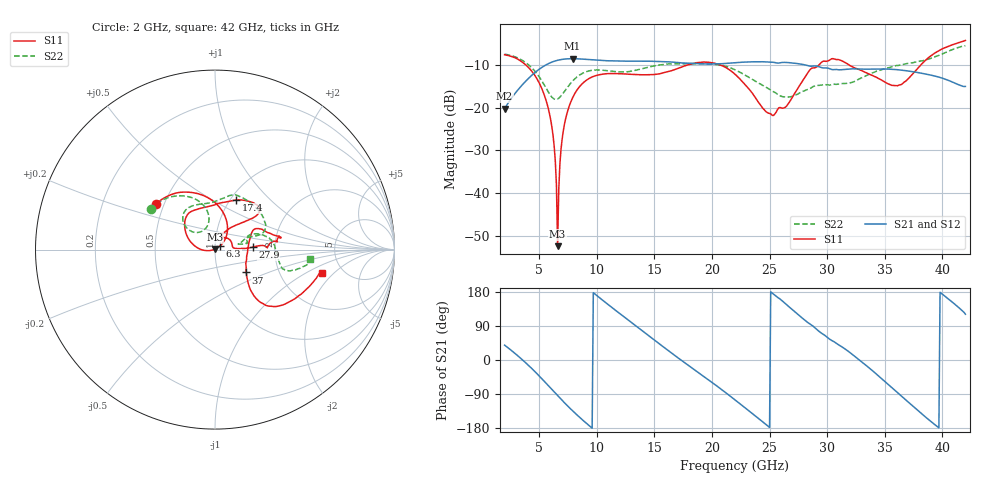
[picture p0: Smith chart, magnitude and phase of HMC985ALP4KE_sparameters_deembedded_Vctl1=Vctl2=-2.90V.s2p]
!s2p File: Measurements: S11, S21, S12, S22
# GHz S dB R 50.0
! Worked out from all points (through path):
!   401 points, 2 GHz to 42 GHz, reference 50 ohm
!   highest |S21| = -8.54 dB at 7.9 GHz (marker M1); lowest = -20.2 dB at 2 GHz (marker M2)
!   lowest |S11| = -52.4 dB at 6.6 GHz (marker M3), VSWR 1.00, Z = 50 + j0.238 ohm
!   |S11| at or under -10 dB: 3.839 GHz to 17.88 GHz (14.05 GHz wide, 129 % of centre); 20.69 GHz to 29.29 GHz (8.598 GHz wide, 34.4 % of centre); 31.9 GHz to 38.13 GHz (6.234 GHz wide, 17.8 % of centre)
!   |S22| runs from -18.1 to -5.5 dB; largest |S21 - S12| = 0.0006
!   S11 on the Smith chart (normalised r, x): 2 GHz: 0.45, +0.28; 6.3 GHz: 1.06, +0.04; 17.4 GHz: 1.06, +0.65; 27.9 GHz: 1.53, +0.04; 37 GHz: 1.36, -0.36; 42 GHz: 3.49, -1.46
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2  -7.62 142.5  -20.23 39.2  -20.22 39.2  -7.48 148.0
5  -14.20 73.6  -11.01 -42.1  -11.00 -42.1  -12.78 102.2
5.8  -20.27 49.5  -9.70 -67.8  -9.70 -67.8  -16.36 103.8
6.3  -28.93 36.4  -9.15 -84.2  -9.16 -84.2  -17.97 117.3
6.4  -32.43 34.9  -9.06 -87.4  -9.07 -87.4  -18.07 120.8
6.6  -52.40 96.2  -8.91 -93.9  -8.93 -93.9  -17.98 127.7
6.8  -33.14 -169.4  -8.80 -100.3  -8.81 -100.3  -17.53 133.7
7.1  -25.34 -174.7  -8.66 -109.8  -8.67 -109.8  -16.54 139.8
7.9  -17.70 165.5  -8.54 -134.0  -8.54 -134.0  -13.78 142.2
8.7  -14.50 149.8  -8.63 -156.4  -8.63 -156.4  -12.06 136.1
12.3  -12.08 118.3  -9.11 115.4  -9.11 115.4  -11.65 97.5
15.4  -12.11 91.4  -9.20 43.3  -9.19 43.3  -10.03 73.8
17.4  -10.46 67.1  -9.53 -1.8  -9.54 -1.8  -9.72 64.1
22  -12.16 41.7  -9.48 -105.2  -9.48 -105.3  -11.14 18.8
25.2  -21.72 58.2  -9.37 177.3  -9.37 177.3  -16.05 16.8
27.9  -13.57 3.8  -9.89 109.1  -9.90 109.1  -16.17 11.2
28.7  -10.73 2.1  -10.30 91.1  -10.30 91.1  -15.19 11.4
32.4  -10.74 21.7  -10.93 9.4  -10.93 9.4  -13.83 22.7
35.4  -14.53 6.9  -10.99 -67.0  -10.99 -67.1  -10.62 14.3
37  -13.33 -36.3  -11.41 -110.0  -11.41 -110.0  -9.66 5.7
39.6  -6.83 -44.2  -12.78 -176.7  -12.78 -176.7  -7.87 -16.3
42  -4.28 -12.4  -15.03 120.8  -15.04 120.7  -5.51 -6.0
